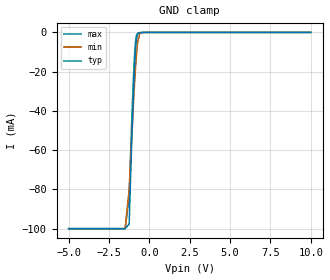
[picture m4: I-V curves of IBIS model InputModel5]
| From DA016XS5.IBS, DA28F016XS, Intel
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|**********************Input Model 5***************************************
[Model]   InputModel5
Model_type   Input
|   for CLK, ADV#
Vinl = 0.8V
Vinh = 2.0V
| Variable   typ   min   max
C_comp   5.61p   NA   7.6p
[Voltage Range]   5.0V   4.5V   5.5V
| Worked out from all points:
|   GND clamp passes 1 mA (typ) near -0.72 V on its own axis
[GND_clamp]
|Voltage I(typ)   I(min)   I(max)
-5V       -99.95mA   -99.95mA   -99.95mA
-1.5V     -99.95mA   -99.95mA   -99.95mA
-1.25V    -97.64mA   -79.9mA    -84.01mA
-1.1V     -58.11mA   -54.7mA    -47.43mA
-950mV    -23.92mA   -31.14mA   -16.55mA
-900mV    -14.92mA   -23.99mA   -9.076mA
-850mV    -8mA       -17.45mA   -4.015mA
-750mV    -1.44mA    -7.157mA   -647.1uA
-700mV    -605.7uA   -3.834mA   -369.1uA
-600mV    -180.3uA   -787uA     -145.6uA
-500mV    -45.79uA   -164.1uA   -31.18uA
10V       0A         0A         0A
[POWER_clamp]
| Input buffer circuits of this product do not intrinsically
| require a [POWER_clamp] definition.  This zero current
| [POWER_clamp] is provided for compatibility with some ibis
| parsers.
|   Voltage  I(typ)   I(min)   I(max)
-5V       0A         0A         0A
-4.75V    0A         0A         0A
9.75V     0A         0A         0A
10V       0A         0A         0A
